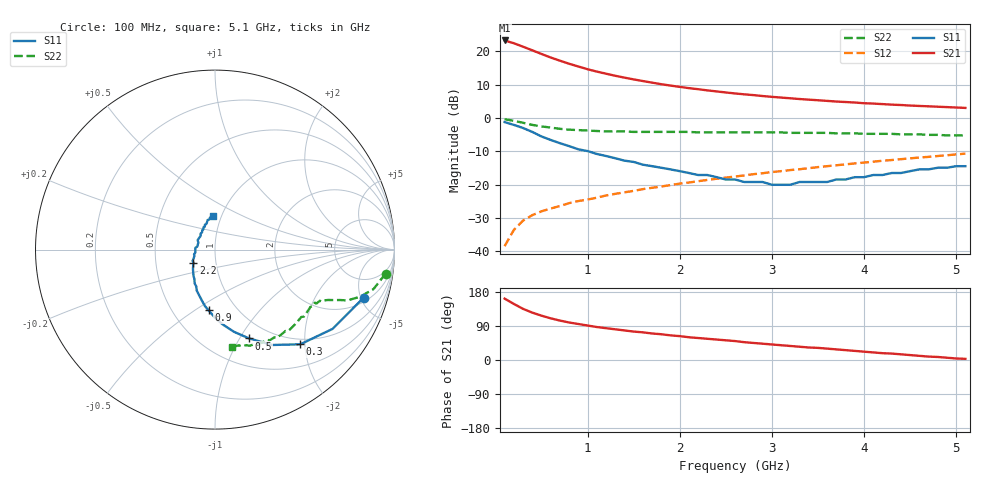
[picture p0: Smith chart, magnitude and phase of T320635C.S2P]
!AT-32063
!S PARAMETERS per side at Vce=5 V  Ic=5mA.  LAST UPDATED 08-19-96
# ghz s ma r 50
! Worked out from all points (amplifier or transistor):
!   51 points, 100 MHz to 5.1 GHz, reference 50 ohm
!   highest |S21| = 23.3 dB at 100 MHz (marker M1)
!   |S21| within 3 dB of that: start of sweep to 404.5 MHz
!   unconditionally stable (mu >= 1): 1.18 GHz to 3.897 GHz; 3.904 GHz to 4.061 GHz
!   at 900 MHz: K = 0.88, MSG = 20.2 dB, |S12| = -24.9 dB
!   at 2.6 GHz: K = 1.10, MAG = 10.6 dB, |S12| = -17.5 dB
!   at 5.1 GHz: K = 0.92, MSG = 6.9 dB, |S12| = -10.7 dB
!   S11 on the Smith chart (normalised r, x): 100 MHz: 2.38, -5.27; 300 MHz: 0.90, -1.91; 500 MHz: 0.80, -1.10; 900 MHz: 0.75, -0.57; 2.2 GHz: 0.78, -0.11; 5.1 GHz: 0.91, +0.36
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0.1  0.87 -18.0  14.58 162.0  0.012 80.0  0.96 -8.0
0.2  0.79 -34.0  13.25 148.0  0.021 72.0  0.91 -14.0
0.3  0.71 -48.0  11.75 135.0  0.029 66.0  0.85 -18.0
0.4  0.62 -59.0  10.38 125.0  0.035 63.0  0.79 -21.0
0.5  0.53 -69.0  9.15 117.0  0.04 60.0  0.75 -22.0
0.6  0.47 -77.0  8.09 110.0  0.044 59.0  0.72 -23.0
0.7  0.42 -84.0  7.25 104.0  0.048 59.0  0.69 -24.0
0.8  0.38 -90.0  6.52 99.0  0.053 59.0  0.67 -25.0
0.9  0.34 -96.0  5.93 95.0  0.057 59.0  0.66 -26.0
1  0.32 -100.0  5.4 91.0  0.06 59.0  0.65 -26.0
1.1  0.29 -105.0  4.98 87.0  0.064 59.0  0.64 -28.0
1.3  0.25 -114.0  4.31 81.0  0.073 59.0  0.63 -29.0
1.4  0.23 -117.0  4.04 78.0  0.077 60.0  0.63 -30.0
1.5  0.22 -121.0  3.8 75.0  0.081 60.0  0.62 -31.0
1.8  0.18 -132.0  3.22 68.0  0.094 59.0  0.62 -33.0
2.1  0.15 -144.0  2.81 60.0  0.108 59.0  0.62 -37.0
2.2  0.14 -149.0  2.71 58.0  0.113 58.0  0.61 -38.0
2.6  0.12 -167.0  2.34 50.0  0.133 57.0  0.61 -42.0
3  0.1 170.0  2.08 41.0  0.155 55.0  0.61 -47.0
3.5  0.11 141.0  1.85 32.0  0.184 51.0  0.6 -53.0
4.3  0.15 112.0  1.59 17.0  0.235 45.0  0.58 -65.0
5.1  0.19 93.0  1.42 3.0  0.293 37.0  0.55 -80.0
